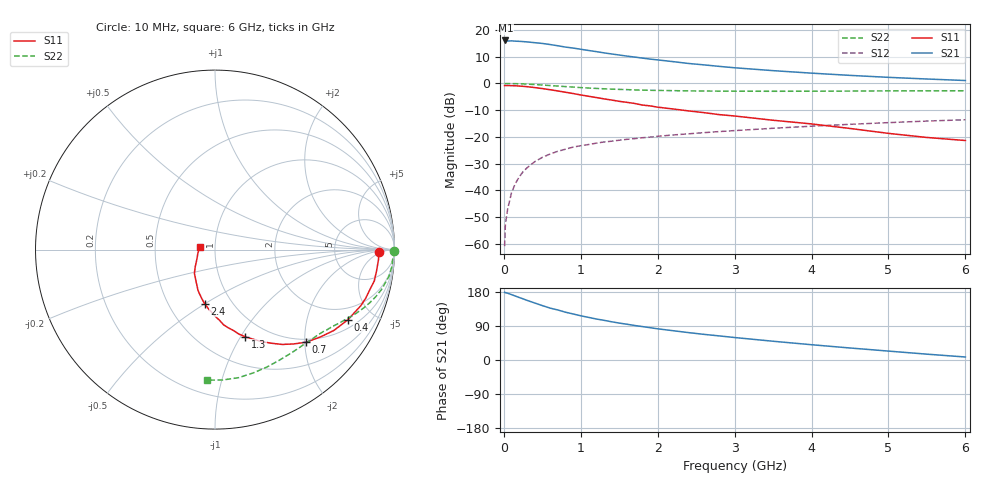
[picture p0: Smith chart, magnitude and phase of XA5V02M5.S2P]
! SIEMENS Discrete & RF Semiconductors
! BFY180
! Si NPN RF Bipolar Junction Transistor in MICRO-X
! VCE = 5 V  IC = 2.5 mA
! Common Emitter S-Parameters:  May  1997
# GHz  S  MA  R  50
!  f  S11  S21  S12  S22
! GHz  MAG  ANG  MAG  ANG  MAG  ANG  MAG  ANG
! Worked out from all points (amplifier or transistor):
!   36 points, 10 MHz to 6 GHz, reference 50 ohm
!   highest |S21| = 16.1 dB at 20 MHz (marker M1)
!   |S21| within 3 dB of that: start of sweep to 935.6 MHz
!   unconditionally stable (mu >= 1): 2.716 GHz to end of sweep
!   at 250 MHz: K = 0.13, MSG = 24.3 dB, |S12| = -33.0 dB
!   at 1.4 GHz: K = 0.72, MSG = 16.3 dB, |S12| = -21.6 dB
!   at 6 GHz: K = 1.06, MAG = 5.8 dB, |S12| = -13.6 dB
!   S11 on the Smith chart (normalised r, x): 10 MHz: 21, -3; 400 MHz: 1.36, -3.55; 700 MHz: 0.94, -2.03; 1.3 GHz: 0.79, -1.05; 2.4 GHz: 0.75, -0.50; 6 GHz: 0.84, +0.03
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0.01  0.9121 -0.7  6.306 178.6  0.0009 71.8  0.9949 -0.3
0.02  0.9123 -1.5  6.373 177.8  0.0023 94.6  0.9953 -0.6
0.05  0.9127 -3.4  6.218 176.2  0.0045 84.1  0.9947 -1.8
0.1  0.9082 -7.3  6.263 172.5  0.009 86.3  0.9905 -3.6
0.15  0.9046 -11.1  6.184 168.8  0.0134 84.1  0.9906 -5.3
0.3  0.8702 -21.1  5.989 157.5  0.0262 76.6  0.971 -10.3
0.4  0.8374 -27.8  5.791 150.5  0.0342 73.7  0.9547 -13.4
0.5  0.8011 -34.2  5.606 143.6  0.0413 69.9  0.9335 -16.3
0.6  0.7631 -39.6  5.349 137.0  0.0477 66.4  0.913 -18.8
0.7  0.7243 -45.4  5.077 132.1  0.0536 63.6  0.893 -21.1
0.8  0.6842 -50.2  4.794 126.2  0.0587 61.1  0.8729 -23.2
0.9  0.6475 -54.7  4.596 121.5  0.0643 58.5  0.8548 -25.2
1.1  0.5752 -63.1  4.14 112.5  0.0718 55.0  0.8207 -28.6
1.3  0.5145 -70.8  3.736 104.8  0.0801 52.1  0.7944 -31.7
1.5  0.4627 -77.1  3.403 97.4  0.0866 50.0  0.7735 -34.5
1.7  0.4218 -83.5  3.118 91.1  0.0927 48.1  0.7559 -37.2
2.2  0.3327 -96.2  2.558 77.3  0.1085 44.2  0.7325 -43.8
2.4  0.3063 -101.0  2.365 72.3  0.1139 43.0  0.7252 -46.2
3.5  0.2046 -121.2  1.735 49.5  0.1448 35.6  0.713 -59.8
4.5  0.1436 -139.7  1.415 31.7  0.1718 28.6  0.7193 -72.7
5.5  0.0974 -168.1  1.21 15.4  0.1975 21.0  0.7278 -86.7
6  0.0854 168.8  1.134 7.9  0.209 16.9  0.7289 -93.7
